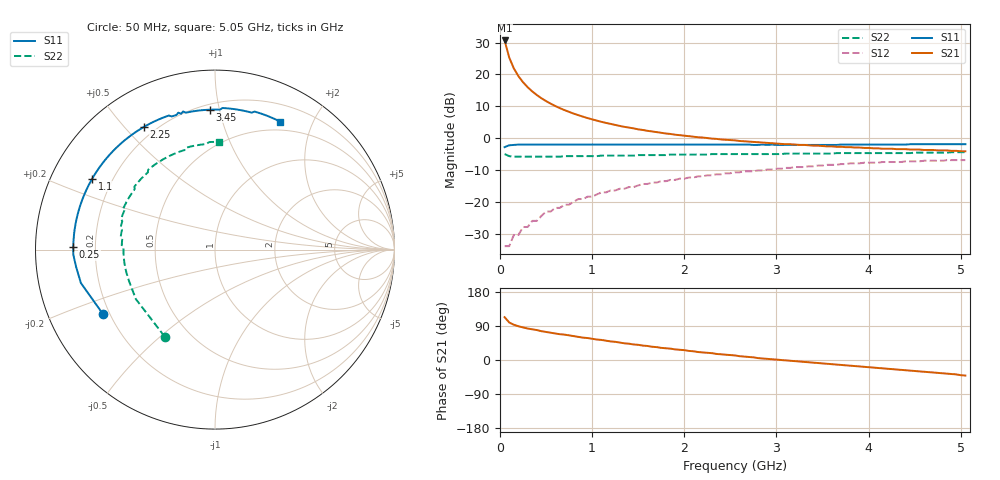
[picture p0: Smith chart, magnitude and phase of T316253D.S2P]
!AT-31625
!S-PARAMETERS at Vce=3.0 V  Ic=200 mA.  LAST UPDATED 08-05-96
# ghz s ma r 50
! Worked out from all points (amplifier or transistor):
!   101 points, 50 MHz to 5.05 GHz, reference 50 ohm
!   highest |S21| = 30.7 dB at 50 MHz (marker M1)
!   |S21| within 3 dB of that: start of sweep to 77.95 MHz
!   unconditionally stable (mu >= 1): 377.9 MHz to 471.1 MHz; 509 MHz to 1.74 GHz; 1.763 GHz to 1.925 GHz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
!   at 850 MHz: K = 1.03, MAG = 12.2 dB, |S12| = -19.2 dB
!   at 2.55 GHz: K = 0.97, MSG = 5.0 dB, |S12| = -10.8 dB
!   at 5.05 GHz: K = 0.98, MSG = 1.4 dB, |S12| = -6.9 dB
!   S11 on the Smith chart (normalised r, x): 50 MHz: 0.17, -0.26; 250 MHz: 0.12, +0.01; 1.1 GHz: 0.13, +0.26; 2.25 GHz: 0.16, +0.57; 3.45 GHz: 0.24, +0.94; 5.05 GHz: 0.39, +1.56
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0.05  0.72 -150.0  34.19 113.0  0.02 40.0  0.56 -120.0
0.1  0.77 -166.0  18.43 99.0  0.02 42.0  0.52 -148.0
0.15  0.78 -173.0  12.45 93.0  0.03 48.0  0.51 -160.0
0.2  0.79 -178.0  9.39 89.0  0.03 53.0  0.51 -165.0
0.25  0.79 179.0  7.54 86.0  0.04 57.0  0.51 -169.0
0.3  0.79 177.0  6.3 83.0  0.04 59.0  0.51 -172.0
0.35  0.79 174.0  5.41 81.0  0.05 61.0  0.51 -173.0
0.4  0.79 172.0  4.74 79.0  0.05 62.0  0.51 -175.0
0.45  0.79 171.0  4.22 76.0  0.06 63.0  0.51 -177.0
0.55  0.79 167.0  3.47 72.0  0.07 64.0  0.51 -179.0
0.65  0.79 164.0  2.95 68.0  0.08 64.0  0.51 179.0
0.8  0.79 159.0  2.42 63.0  0.1 63.0  0.52 177.0
0.9  0.79 156.0  2.17 59.0  0.11 62.0  0.52 175.0
1.1  0.79 150.0  1.8 53.0  0.14 60.0  0.53 172.0
1.35  0.79 144.0  1.5 44.0  0.16 56.0  0.53 169.0
1.75  0.79 133.0  1.21 32.0  0.21 49.0  0.54 164.0
2.25  0.79 120.0  1 19.0  0.26 41.0  0.55 156.0
2.55  0.79 112.0  0.92 12.0  0.29 35.0  0.56 152.0
3.4  0.78 93.0  0.76 -7.0  0.36 19.0  0.57 136.0
3.45  0.78 92.0  0.76 -8.0  0.37 18.0  0.57 135.0
4.25  0.79 77.0  0.68 -24.0  0.42 1.0  0.58 113.0
5.05  0.8 63.0  0.62 -41.0  0.45 -16.0  0.6 88.0
